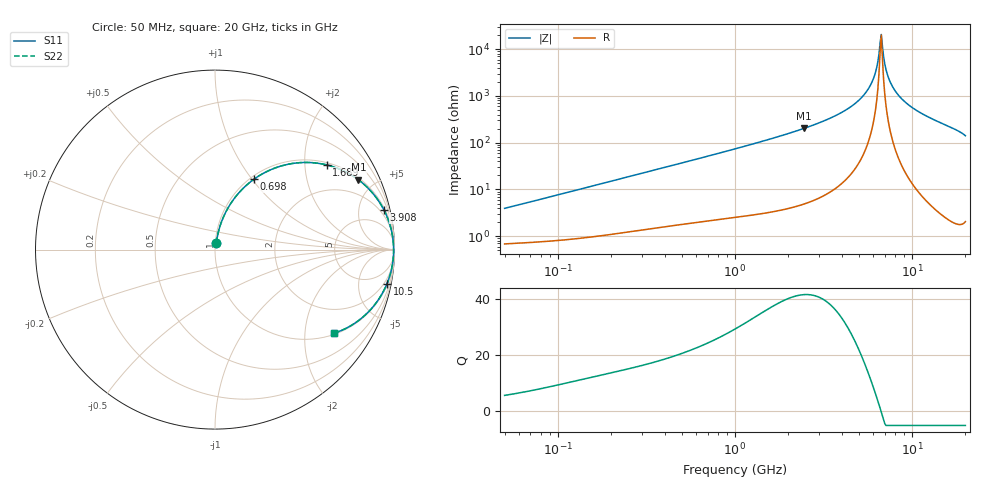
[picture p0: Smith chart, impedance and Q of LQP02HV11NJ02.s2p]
!Murata Part Number: LQP02HV11NJ02
!These Parameters are Measured in Series Mode Connection
!  o--[Z]--o
!Port1  Port2
!  o-------o
!Freq. Start=50[MHz] Stop=20[GHz], 401[Steps]
# Hz S RI R 50
!Freq.(Hz) S11(Real) S11(Imag) S21(Real) S21(Imag) S12(Real) S12(Imag) S22(Real) S22(Imag)
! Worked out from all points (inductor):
!   401 points, 50 MHz to 20 GHz, reference 50 ohm
!   read as one part in series: L = 12.3 nH near 51.52 MHz
!   highest Q = 41.5 at 2.456 GHz (marker M1), where L = 13.1 nH
!   self-resonance near 6.602 GHz
!   S11 on the Smith chart (normalised r, x): 50 MHz: 1.01, +0.08; 698 MHz: 1.04, +1.02; 1.689 GHz: 1.07, +2.58; 3.908 GHz: 1.25, +8.45; 10.5 GHz: 1, -10; 20 GHz: 1.04, -2.82
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5e7  0.00827 0.0383  0.9917 -0.0383  0.9917 -0.0383  0.00827 0.0383
1.364002e8  0.0193 0.1003  0.9807 -0.1003  0.9807 -0.1003  0.0193 0.1003
3.721004e8  0.0823 0.2484  0.9177 -0.2484  0.9177 -0.2484  0.0823 0.2484
6.980337e8  0.2173 0.3923  0.7827 -0.3923  0.7827 -0.3923  0.2173 0.3923
1e9  0.3569 0.4623  0.6431 -0.4623  0.6431 -0.4623  0.3569 0.4623
1.689197e9  0.6223 0.4718  0.3777 -0.4718  0.3777 -0.4718  0.6223 0.4718
2.456456e9  0.7988 0.3891  0.2012 -0.3891  0.2012 -0.3891  0.7988 0.3891
2.728004e9  0.8392 0.3555  0.1608 -0.3555  0.1608 -0.3555  0.8392 0.3555
3.908127e9  0.9412 0.221  0.0588 -0.221  0.0588 -0.221  0.9412 0.221
4.89267e9  0.9771 0.1296  0.0229 -0.1296  0.0229 -0.1296  0.9771 0.1296
5.683258e9  0.9902 0.0677  0.00977 -0.0677  0.00977 -0.0677  0.9902 0.0677
6.125241e9  0.9937 0.0365  0.00627 -0.0365  0.00627 -0.0365  0.9937 0.0365
6.311513e9  0.9946 0.024  0.00543 -0.024  0.00543 -0.024  0.9946 0.024
6.503449e9  0.9951 0.0115  0.00491 -0.0115  0.00491 -0.0115  0.9951 0.0115
6.701223e9  0.9953 -0.001  0.00471 0.001  0.00471 0.001  0.9953 -0.001
6.802353e9  0.9953 -0.00726  0.00473 0.00726  0.00473 0.00726  0.9953 -0.00726
7.114996e9  0.9947 -0.0261  0.00527 0.0261  0.00527 0.0261  0.9947 -0.0261
7.442007e9  0.9935 -0.0449  0.00653 0.0449  0.00653 0.0449  0.9935 -0.0449
8.516016e9  0.9852 -0.1017  0.0148 0.1017  0.0148 0.1017  0.9852 -0.1017
1.050288e10  0.958 -0.1905  0.042 0.1905  0.042 0.1905  0.958 -0.1905
1.573793e10  0.8406 -0.361  0.1594 0.361  0.1594 0.361  0.8406 -0.361
2e10  0.663 -0.4655  0.337 0.4655  0.337 0.4655  0.663 -0.4655
